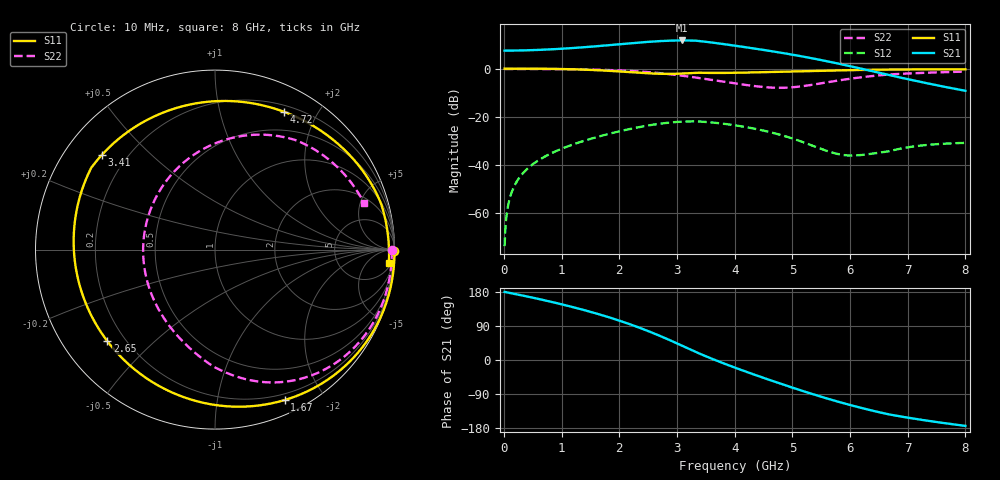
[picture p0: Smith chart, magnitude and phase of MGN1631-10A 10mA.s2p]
! Port[1] = GATE
! Port[2] = DRAIN
! [Type]  S-parameter s2p file touchstone ver. 1.0
! [Object]  MGN1631-10A
! [Bias]  10 mA
! [Version]  1.0
! [Date]  Thu May 19 10:54:03 2026
! [Source]  This file was created in JSC "ICC Milandr".
! [Disclaimer] Property of JSC "ICC Milandr". Unauthorized reproduction and/or distribution is strictly prohibited.
!  The file and the data are provided "AS IS" and with all faults and disclaim all warranties, express and implied, including
!  without limitation any implied warranties of merchantability, fitness for a particular purpose.
!  JSC "ICC Milandr" assumes no liability for:
!  1) the accuracy of the data provided;
!  2) the proper functioning of this data;
!  3) infringement of patents, copyrights or intellectual property rights resulting from the use of this data.
!  JSC "ICC Milandr" reserves the right to make changes to the products and the data without prior notice.
!  Please, be aware that your receipt and use of the file provided shall serve as acceptance of these terms and conditions.
!  If you do not accept these terms, you should return or destroy this file and any other accompanying information immediately.
# Hz S MA R 12.5
! freq  S11mag  S11ang  S21mag  S21ang  S12mag  S12ang  S22mag  S22ang
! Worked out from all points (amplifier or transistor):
!   800 points, 10 MHz to 8 GHz, reference 12.5 ohm
!   highest |S21| = 11.7 dB at 3.09 GHz (marker M1)
!   |S21| within 3 dB of that: 1.281 GHz to 4.242 GHz (2.96 GHz wide, 107 % of centre)
!   unconditionally stable (mu >= 1): 4.763 GHz to 6.954 GHz
!   at 1.34 GHz: K = 0.25, MSG = 19.6 dB, |S12| = -30.3 dB
!   at 4.01 GHz: K = 0.67, MSG = 16.5 dB, |S12| = -23.6 dB
!   at 8 GHz: K = 0.75, MSG = 10.8 dB, |S12| = -30.8 dB
!   S11 on the Smith chart (normalised r, x): 10 MHz: open; 1.67 GHz: 0.14, -1.56; 2.65 GHz: 0.13, -0.36; 3.41 GHz: 0.11, +0.36; 4.72 GHz: 0.27, +1.58; 8 GHz: 8, -23
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1e7  1 -0.3  2.373 179.7  0.0002047 86.0  0.9851 -0.2
1.1e8  1.001 -3.5  2.376 176.7  0.002239 86.7  0.9855 -2.1
3.1e8  1.001 -10.1  2.397 170.5  0.006353 81.6  0.9858 -5.9
8.9e8  0.9891 -30.3  2.552 151.0  0.01909 64.7  0.9807 -17.4
1.35e9  0.9586 -49.3  2.771 133.3  0.03065 49.1  0.9665 -27.5
1.67e9  0.9236 -65.2  2.972 119.6  0.03971 36.8  0.9483 -35.2
1.97e9  0.8813 -83.1  3.194 105.4  0.04895 23.9  0.9227 -43.1
2.25e9  0.8375 -103.4  3.417 90.7  0.05802 10.4  0.8887 -51.4
2.65e9  0.7874 -139.7  3.711 67.0  0.07039 -11.8  0.8188 -64.5
2.68e9  0.7853 -142.7  3.729 65.1  0.07122 -13.6  0.8125 -65.6
2.88e9  0.7798 -164.0  3.823 52.0  0.07602 -26.0  0.7669 -72.9
3.09e9  0.792 173.0  3.86 37.6  0.07936 -39.8  0.7144 -80.8
3.28e9  0.8169 152.7  3.83 24.3  0.0805 -52.6  0.6658 -88.4
3.41e9  0.8223 140.3  3.728 15.5  0.07958 -60.6  0.6322 -93.6
3.68e9  0.8155 118.4  3.4 -1.3  0.07465 -74.2  0.5653 -104.7
4.01e9  0.8222 96.5  2.999 -20.5  0.06641 -88.4  0.4935 -121.4
4.35e9  0.8377 78.7  2.614 -39.2  0.05638 -100.5  0.4341 -144.0
4.72e9  0.8585 63.5  2.228 -58.7  0.04448 -110.3  0.4012 -175.5
5.34e9  0.8958 44.2  1.646 -89.5  0.02538 -113.9  0.462 128.1
5.93e9  0.9287 30.0  1.177 -115.8  0.01586 -87.1  0.601 87.8
6.67e9  0.9602 15.3  0.7404 -143.5  0.01904 -57.6  0.7575 53.6
8e9  0.9714 -4.4  0.347 -174.0  0.02873 -79.6  0.8692 17.5
